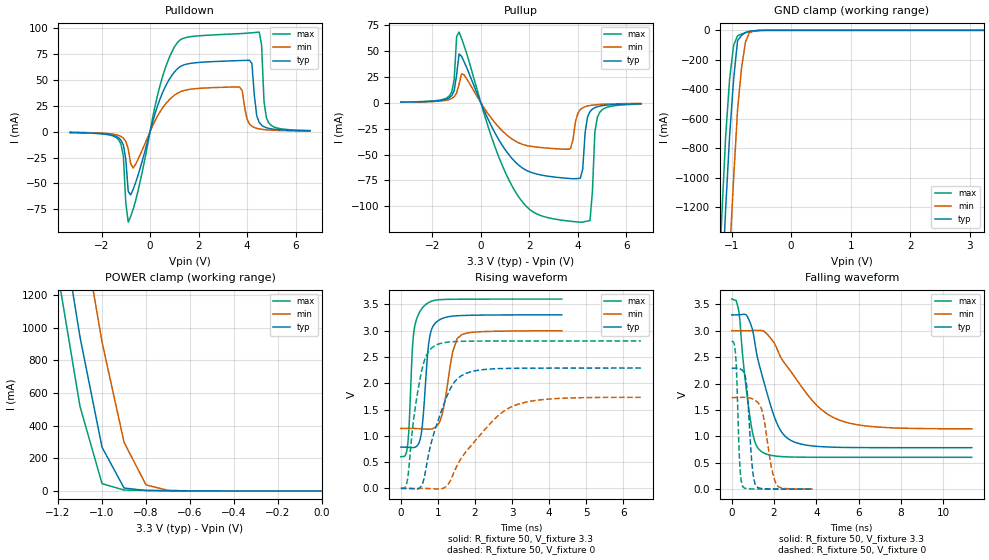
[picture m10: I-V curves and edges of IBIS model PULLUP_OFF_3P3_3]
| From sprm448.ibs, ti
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|   Model Cell PULLUP_OFF_3P3
|PULLUP_OFF_3P3
[Model]   PULLUP_OFF_3P3_3
Model_type   I/O
Polarity   Non-Inverting
Enable   Active-Low
Vinl =  0.8v
Vinh =  2v
Cref =  15.0000pF
Rref =  100.0000M
Vref =  0V
Vmeas =  1.65
C_comp   2.5107p   2.136p   3.1702p
[Model Spec]
Vinl   0.8v   0.8v   0.8v
Vinh   2v   2v   2v
[Temperature Range]   25   125   -40
[Voltage Range]   3.3   3   3.6
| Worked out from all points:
|   slope of the pulldown table from 0 to 0.495 V, typ, clamps not added: 13.6 ohm
|   slope of the pullup table from 0 to 0.495 V, typ, clamps not added: 19.6 ohm
|   GND clamp passes 1 mA (typ) near -0.55 V on its own axis
|   POWER clamp passes 1 mA (typ) near -0.67 V on its own axis
|   rising waveform, R_fixture 50, V_fixture 3.3: 20-80 % time 168ps typ, 264ps min, 133ps max; typ from 0.785 V to 3.3 V
|   rising waveform, R_fixture 50, V_fixture 0: 20-80 % time 594ps typ, 1.17ns min, 327ps max; typ from 0 V to 2.29 V
|   falling waveform, R_fixture 50, V_fixture 3.3: 20-80 % time 1.01ns typ, 2.05ns min, 501ps max; typ from 3.3 V to 0.785 V
|   falling waveform, R_fixture 50, V_fixture 0: 20-80 % time 227ps typ, 418ps min, 144ps max; typ from 2.29 V to 0.001 V
[POWER_clamp]
|   voltage   I(typ)   I(min)   I(max)
-3.3V     22.13A     22.81A     21.76A
-1.2V     1.777A     2.558A     1.326A
-1.167V   1.499A     2.271A     1.056A
-1.133V   1.22A      1.985A     786.7mA
-1.1V     941.2mA    1.698A     517.2mA
-1.067V   716.7mA    1.436A     359.6mA
-1.033V   492.2mA    1.174A     202mA
-1V       267.6mA    912.2mA    44.37mA
-900mV    17.85mA    298.1mA    5.46mA
-800mV    2.603mA    36.52mA    3.101mA
-700mV    1.197mA    3.396mA    1.507mA
-11.55fV  42.09pA    6.147nA    541.8fA
[Pulldown]
|   voltage   I(typ)   I(min)   I(max)
-3.3V     -841.7uA   -670.2uA   -911.7uA
-1.3V     -5.852mA   -3.631mA   -7.719mA
-1.1V     -12.99mA   -6.251mA   -23.51mA
-900mV    -57.7mA    -16.72mA   -87.34mA
-700mV    -55.82mA   -35.09mA   -75.1mA
1.1V      59.92mA    36.57mA    85.06mA
3.7V      68.51mA    42.92mA    94.48mA
4.1V      68.79mA    7.362mA    95.13mA
4.5V      8.911mA    2.645mA    95.99mA
4.7V      4.671mA    1.979mA    28.88mA
4.9V      3.124mA    1.577mA    8.243mA
6.6V      798.5uA    571.1uA    1.034mA
[Pullup]
|   voltage   I(typ)   I(min)   I(max)
-3.3V     669.2uA    562.7uA    746.5uA
-1.3V     4.957mA    3.264mA    6.677mA
-1.1V     12mA       5.961mA    22.79mA
-1V       26.99mA    9.54mA     64.01mA
-900mV    47.32mA    18.06mA    68.43mA
1.5V      -59.02mA   -37.99mA   -88.89mA
3.7V      -73.26mA   -44.09mA   -114.6mA
4.1V      -72.87mA   -6.563mA   -115.5mA
4.5V      -8.455mA   -2.591mA   -113.8mA
4.7V      -4.668mA   -1.97mA    -28.57mA
4.9V      -3.189mA   -1.585mA   -9.198mA
6.6V      -843.6uA   -589.3uA   -1.225mA
[GND_clamp]
|   voltage   I(typ)   I(min)   I(max)
-3.3V     -22.45A    -23.24A    -22.02A
-1.233V   -2.371A    -3.249A    -1.858A
-1.167V   -1.783A    -2.654A    -1.277A
-1.1V     -1.21A     -2.069A    -720.1mA
-1.033V   -714.5mA   -1.52A     -330.7mA
-966.7mV  -334.2mA   -1.01A     -102.9mA
-900mV    -69.1mA    -538.9mA   -36.77mA
-833.3mV  -34.65mA   -254mA     -25.31mA
-766.7mV  -14mA      -79.21mA   -15.48mA
-700mV    -7.158mA   -14.43mA   -7.256mA
-433.3mV  -74.68uA   -266.3uA   -24.2uA
3.233V    39.36pA    1.428uA    458.9fA
[Ramp]
| variable   typ   min   max
dV/dt_f   1.515963/1.010838n   1.120146/2.051459n   1.80798/0.5017609n
dV/dt_r   1.381504/0.5947873n   1.048334/1.177938n   1.690692/0.3269337n
R_load = 50
[Rising Waveform]
R_fixture = 50
V_fixture = 3.3
V_fixture_min = 3
V_fixture_max = 3.6
|   time   V(typ)   V(min)   V(max)
0s        785.3mV    1.141V     603.3mV
184ps     782.3mV    1.142V     826.1mV
368ps     780mV      1.14V      3.061V
528ps     953.5mV    1.135V     3.378V
632ps     1.644V     1.13V      3.471V
784ps     2.906V     1.126V     3.546V
1.04ns    3.204V     1.26V      3.588V
1.4ns     3.276V     2.6V       3.596V
1.648ns   3.287V     2.925V     3.597V
4.344ns   3.299V     2.997V     3.6V
[Rising Waveform]
R_fixture = 50
V_fixture = 0
V_fixture_min = 0
V_fixture_max = 0
|   time   V(typ)   V(min)   V(max)
0s        58.79pV    18.53nV    1.601pV
184ps     520.9uV    135.3uV    187mV
352ps     -8.159mV   298.5uV    1.351V
560ps     53.44mV    433.4uV    2.227V
704ps     484.4mV    -911.2uV   2.548V
920ps     1.109V     -8.243mV   2.714V
1.24ns    1.746V     48.29mV    2.779V
1.552ns   2.1V       481.7mV    2.795V
2.944ns   2.283V     1.539V     2.802V
6.48ns    2.288V     1.732V     2.803V
[Falling Waveform]
R_fixture = 50
V_fixture = 3.3
V_fixture_min = 3
V_fixture_max = 3.6
|   time   V(typ)   V(min)   V(max)
0s        3.3V       3V         3.6V
352ps     3.303V     3V         3.328V
768ps     3.248V     3.002V     1.647V
1.04ns    2.914V     3.004V     976.1mV
1.448ns   2.139V     3.002V     701.4mV
2.192ns   1.199V     2.609V     622.5mV
3.04ns    881.7mV    2.09V      607.2mV
4.208ns   805.7mV    1.518V     603.8mV
5.4ns     790.1mV    1.267V     603.3mV
11.35ns   785.4mV    1.144V     603.3mV
[Falling Waveform]
R_fixture = 50
V_fixture = 0
V_fixture_min = 0
V_fixture_max = 0
|   time   V(typ)   V(min)   V(max)
0s        2.289V     1.735V     2.803V
184ps     2.292V     1.736V     2.546V
392ps     2.279V     1.739V     397.4mV
536ps     2.237V     1.74V      43.19mV
712ps     1.945V     1.736V     10.55mV
952ps     507.6mV    1.713V     5.06mV
1.144ns   67.04mV    1.672V     3.482mV
1.472ns   10.51mV    1.431V     2.14mV
2.144ns   2.984mV    75.92mV    826.8uV
3.832ns   727uV      3.01mV     137.4uV
